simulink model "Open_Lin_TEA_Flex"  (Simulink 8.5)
settings: Solver=ode113  StartTime=0.0  StopTime=100000  RelTol=1e-3
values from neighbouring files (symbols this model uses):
  Kpqr = lqr(sys,Q0,R0)    [des.m]
  wo = 0.0011    [start.m]    (also in start1.m; start2.m; start3.m)
undefined symbols (not defined in the file or in its folder): Af, Bf, Cf, Df

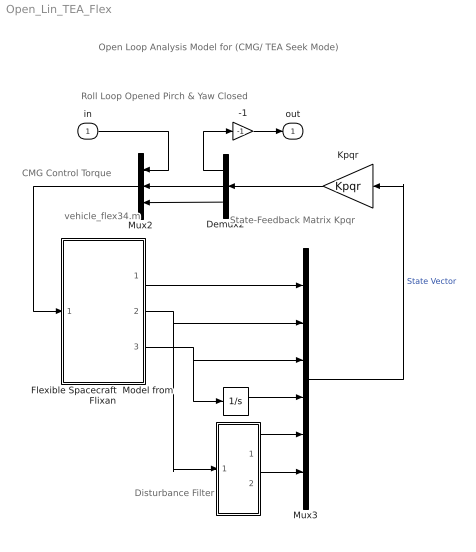
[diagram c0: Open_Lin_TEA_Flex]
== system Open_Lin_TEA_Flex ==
  note: Open Loop Analysis Model for (CMG/ TEA Seek Mode)
  note: CMG Control Torque
  note: Disturbance Filter
  note: State-Feedback Matrix Kpqr
  note: Roll Loop Opened Pirch & Yaw Closed
  note: vehicle_flex34.m
  in : Inport  PortDimensions=1
  " " : Subsystem
  "  " : Integrator
  -1 : Gain  Gain=-1
  Demux2 : Demux  Outputs=3
  Flexible Spacecraft  Model from Flixan : Subsystem
  Kpqr : Gain  Gain=Kpqr  Multiplication=Matrix(K*u)
  Mux2 : Mux  Inputs=3
  Mux3 : Mux  Inputs=[3, 3, 3, 3, 1, 1]
  out : Outport
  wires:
  "  "/1 -> Mux3/4
  Mux3/1 -> Kpqr/1  "State Vector"
  " "/1(a1) -> Mux3/5
  " "/2(a2) -> Mux3/6
  Flexible Spacecraft  Model from Flixan/1(w-lv) -> Mux3/1
  Mux2/1 -> Flexible Spacecraft  Model from Flixan/1(Tcmg)
  Kpqr/1 -> Demux2/1
  -1/1 -> out/1
  Flexible Spacecraft  Model from Flixan/2(att-lv) -> Mux3/2, " "/1(the)
  Flexible Spacecraft  Model from Flixan/3("Hcmg ") -> Mux3/3, "  "/1
  Demux2/3 -> Mux2/3
  Demux2/2 -> Mux2/2
  in/1 -> Mux2/1
  Demux2/1 -> -1/1

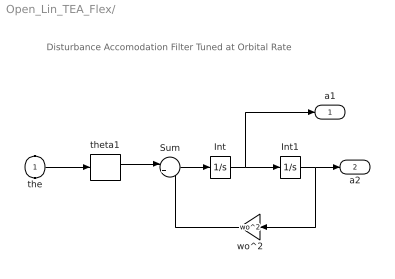
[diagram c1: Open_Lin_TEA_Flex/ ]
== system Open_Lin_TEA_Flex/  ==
  note: Disturbance Accomodation Filter Tuned at Orbital Rate
  the : Inport
  Int : Integrator
  Int1 : Integrator
  Sum : Sum  Inputs=|+-
  theta1 : Selector  InputPortWidth=3  Indices=[2]
  wo^2 : Gain  Gain=wo^2
  a1 : Outport
  a2 : Outport  Port=2
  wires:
  Int/1 -> Int1/1, a1/1
  Sum/1 -> Int/1
  Int1/1 -> wo^2/1, a2/1
  wo^2/1 -> Sum/2
  theta1/1 -> Sum/1
  the/1 -> theta1/1

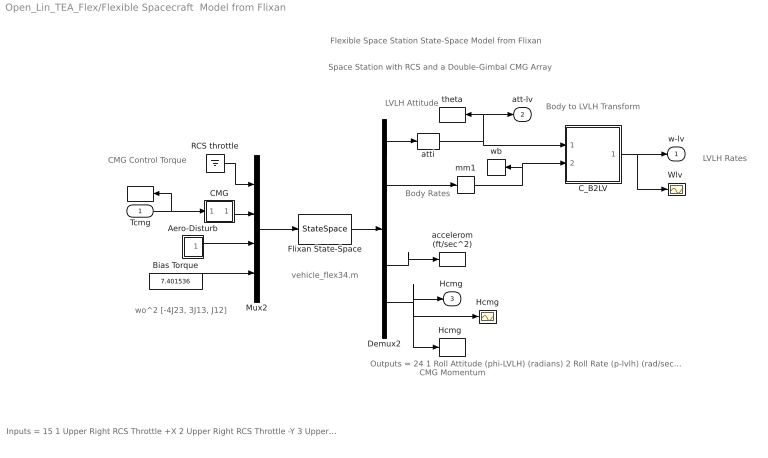
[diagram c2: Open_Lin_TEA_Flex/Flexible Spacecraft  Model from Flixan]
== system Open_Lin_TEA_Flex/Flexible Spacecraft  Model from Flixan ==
  note: Outputs = 24 1 Roll Attitude (phi-LVLH) (radians) 2 Roll Rate (p-lvlh) (rad/sec) 3 Pitch Attitude (thet-LVLH) (radians) 4 Pitch Rate (q-lvlh) (rad/sec) 5 Yaw Attitude (psi-LVLH) (radians) 6 Yaw Rate (r-lvlh) (rad/sec) 7 Angle of attack, alfa, (radians) 8 Angle of sideslip, beta, (radian) 9 Change in Altitude, delta-h, (feet) 10 Forward Acceleration (V-dot) (ft/sec) 11 Cross Range Velocity (Vcr) (ft/sec) 12 Rate-Gyro # 1, Roll Rate (Body) (rad/sec) 13 Rate-Gyro # 2, Pitch Rate (Body) (rad/sec) 14 Rate-Gyro # 3, Yaw Rate (Body) (rad/sec) 15 Gyro # 4, Roll Attitude (Body) (radians) 16 Gyro # 5, Pitch Attitude (Body) (radians) 17 Gyro # 6, Yaw Attitude (Body) (radians) 18 Accelerom # 1, (along X), (ft/sec^2) Translat. Accelerat. 19 Accelerom # 2, (along Z), (ft/sec^2) Translat. Accelerat. 20 Accelerom # 3, (along X), (ft/sec^2) Translat. Accelerat. 21 Accelerom # 4, (along Z), (ft/sec^2) Translat. Accelerat. 22 Double Gimbal CMG Momentum Change in X-axis (ft-lb-sec) 23 Double Gimbal CMG Momentum Change in Y-axis (ft-lb-sec) 24 Double Gimbal CMG Momentum Change in Z-axis (ft-lb-sec)
  note: vehicle_flex34.m
  note: CMG Control Torque
  note: Body Rates
  note: Body to LVLH Transform
  note: LVLH Rates
  note: LVLH Attitude
  note: CMG Momentum
  note: Inputs = 15 1 Upper Right RCS Throttle +X 2 Upper Right RCS Throttle -Y 3 Upper Left RCS Throttle +X 4 Upper Left RCS Throttle +Y 5 Lower Right RCS Throttle +X 6 Lower Right RCS Throttle -Y 7 Lower Left RCS Throttle +X 8 Lower Left RCS Throttle +Y 9 Double Gimbal CMG Torque in the X-axis (ft-lb) 10 Double Gimbal CMG Torque in the Y-axis (ft-lb) 11 Double Gimbal CMG Torque in the Z-axis (ft-lb) 12 External Torque Input 1 (ft-lb), direct: 13 External Torque Input 2 (ft-lb), direct: 14 External Torque Input 3 (ft-lb), direct: 15 Ext Torque Direct.=(0.197, -0.5964, -0.7782)
  note: wo^2 [-4J23, 3J13, J12]
  note: Space Station with RCS and a Double-Gimbal CMG Array
  note: Flexible Space Station State-Space Model from Flixan
  Tcmg : Inport  PortDimensions=3
  "   " : ToWorkspace  VariableName=Tcmg  SampleTime=-1
  Aero-Disturb : Subsystem
  Bias Torque : Constant  Value=7.401536
  CMG : Subsystem
  C_B2LV : Subsystem
  Demux2 : Demux  Outputs=[11, 3, 3, 4, 3]
  Flixan State-Space : StateSpace  A=Af  B=Bf  C=Cf  D=Df  X0=0
  Hcmg : Scope
  "Hcmg  " : ToWorkspace  VariableName=Hcmg  SampleTime=-1
  Mux2 : Mux  Inputs=[8, 3, 3, 1]
  RCS throttle : Ground
  "Wlv " : Scope
  accelerom (ft/sec^2) : ToWorkspace  VariableName=accel  SampleTime=-1
  atti : Selector  InputPortWidth=11  Indices=[1 3 5]
  mm1 : Memory
  theta : ToWorkspace  VariableName=theta  SampleTime=-1
  wb : ToWorkspace  VariableName=wb  SampleTime=-1
  w-lv : Outport
  att-lv : Outport  Port=2
  "Hcmg " : Outport  Port=3
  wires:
  C_B2LV/1(wlv) -> w-lv/1, "Wlv "/1
  Demux2/2 -> mm1/1
  atti/1 -> C_B2LV/1(atti), att-lv/1, theta/1
  CMG/1(O) -> Mux2/2
  Aero-Disturb/1(Td) -> Mux2/3
  Tcmg/1 -> "   "/1, CMG/1(I)
  Demux2/4 -> accelerom (ft/sec^2)/1
  Demux2/1 -> atti/1
  Demux2/5 -> "Hcmg  "/1, Hcmg/1, "Hcmg "/1
  RCS throttle/1 -> Mux2/1
  Bias Torque/1 -> Mux2/4
  Flixan State-Space/1 -> Demux2/1
  Mux2/1 -> Flixan State-Space/1
  mm1/1 -> wb/1, C_B2LV/2(wb)

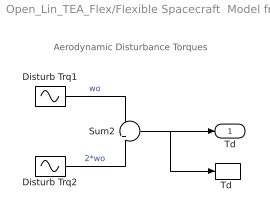
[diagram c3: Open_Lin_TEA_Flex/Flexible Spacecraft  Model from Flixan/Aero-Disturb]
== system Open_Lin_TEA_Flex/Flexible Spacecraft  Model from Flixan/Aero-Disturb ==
  note: Aerodynamic Disturbance Torques
  Disturb Trq1 : Sin  Amplitude=[1, 3, 1]  Bias="[1  8  1]"  Frequency=[wo, wo, wo]  SampleTime=0
  Disturb Trq2 : Sin  Amplitude=[1, 1, 1]*0.5  Frequency=[wo, wo, wo]*2  SampleTime=0
  Sum2 : Sum  Inputs=+|+
  "Td " : ToWorkspace  VariableName=Td  SampleTime=-1
  Td : Outport
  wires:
  Disturb Trq2/1 -> Sum2/2  "2*wo"
  Sum2/1 -> "Td "/1, Td/1
  Disturb Trq1/1 -> Sum2/1  "wo"

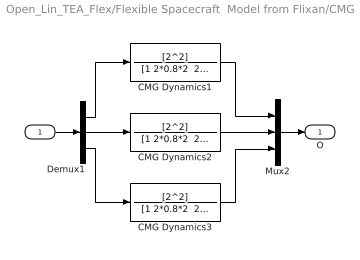
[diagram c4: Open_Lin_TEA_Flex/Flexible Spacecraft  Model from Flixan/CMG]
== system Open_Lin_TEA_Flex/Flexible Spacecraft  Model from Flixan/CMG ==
  I : Inport
  CMG Dynamics1 : TransferFcn  Numerator=[2^2]  Denominator="[1 2*0.8*2  2^2]"
  CMG Dynamics2 : TransferFcn  Numerator=[2^2]  Denominator="[1 2*0.8*2  2^2]"
  CMG Dynamics3 : TransferFcn  Numerator=[2^2]  Denominator="[1 2*0.8*2  2^2]"
  Demux1 : Demux  Outputs=3
  Mux2 : Mux  Inputs=3
  O : Outport
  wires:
  CMG Dynamics2/1 -> Mux2/2
  CMG Dynamics3/1 -> Mux2/3
  CMG Dynamics1/1 -> Mux2/1
  Demux1/2 -> CMG Dynamics2/1
  Demux1/1 -> CMG Dynamics1/1
  Demux1/3 -> CMG Dynamics3/1
  I/1 -> Demux1/1
  Mux2/1 -> O/1

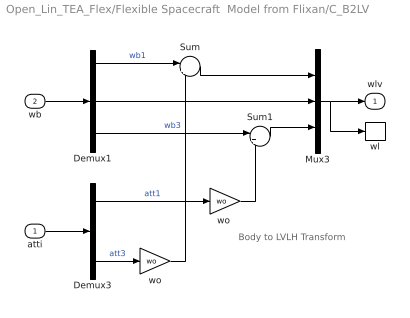
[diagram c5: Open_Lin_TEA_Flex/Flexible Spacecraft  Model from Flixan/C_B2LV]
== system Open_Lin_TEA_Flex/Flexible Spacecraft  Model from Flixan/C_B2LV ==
  note: Body to LVLH Transform
  atti : Inport  PortDimensions=3
  wb : Inport  Port=2  PortDimensions=3
  Demux1 : Demux  Outputs=3
  Demux3 : Demux  Outputs=3
  Mux3 : Mux  Inputs=3
  Sum : Sum  Inputs=|++
  Sum1 : Sum  Inputs=|+-
  wl : ToWorkspace  VariableName=wl  SampleTime=-1
  wo : Gain  Gain=wo
  "wo " : Gain  Gain=wo
  wlv : Outport
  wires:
  Demux1/1 -> Sum/1  "wb1"
  Sum/1 -> Mux3/1
  Demux3/3 -> wo/1  "att3"
  Sum1/1 -> Mux3/3
  atti/1 -> Demux3/1
  wb/1 -> Demux1/1
  Mux3/1 -> wlv/1, wl/1
  Demux3/1 -> "wo "/1  "att1"
  Demux1/2 -> Mux3/2
  wo/1 -> Sum/2
  Demux1/3 -> Sum1/1  "wb3"
  "wo "/1 -> Sum1/2
